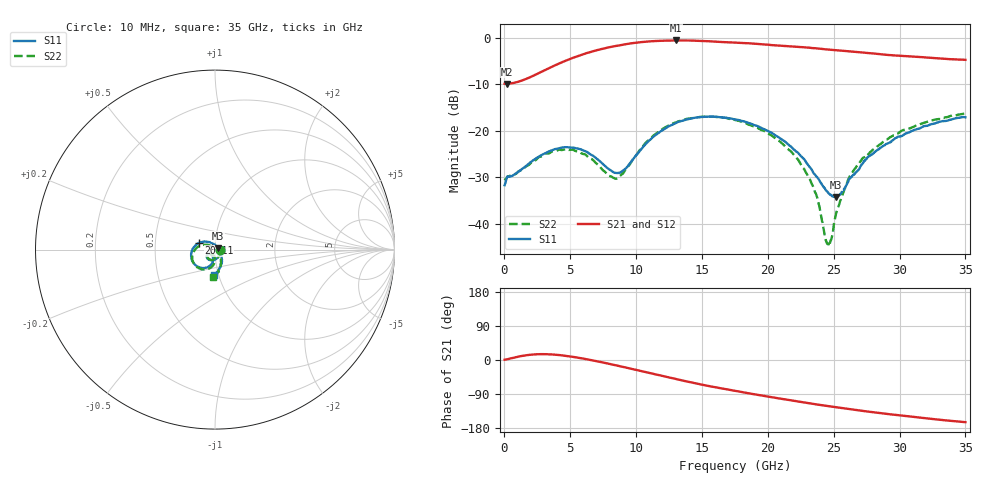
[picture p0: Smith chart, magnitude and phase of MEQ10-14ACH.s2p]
! MARKI MICROWAVE INC.
! Email:  support@markimicrowave.com  Phone:  408-778-4200
! Model Number:  MEQ10-14ACH  Date:  6/18
! Filename:		MEQ10-14ACH.S2P  Version: 1.0
! Description:  2-port S-parameter data for chip equalizer
! Features:		Low Insertion Loss, Excellent Return Loss
! Frequency Measured: 	10 MHz to 35 GHz
!S2P File: Measurements: S11, S21, S12, S22:
# Hz S  dB  R 50
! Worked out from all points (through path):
!   1601 points, 10 MHz to 35 GHz, reference 50 ohm
!   highest |S21| = -0.61 dB at 13 GHz (marker M1); lowest = -9.9 dB at 206.8 MHz (marker M2)
!   group delay of S21, straight-line fit = 16.2 ps
!   lowest |S11| = -34.3 dB at 25.16 GHz (marker M3), VSWR 1.04, Z = 51.7 + j0.915 ohm
!   |S11| at or under -10 dB: start of sweep to end of sweep
!   |S22| runs from -44.9 to -16.3 dB; largest |S21 - S12| = 0.0061
!   S11 on the Smith chart (normalised r, x): 10 MHz: 1.05, -0.00; 20.11 GHz: 0.83, +0.06; 35 GHz: 0.96, -0.27
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1e7  -31.76 -2.9  -9.92 0.7  -9.96 0.0  -30.69 -5.9
2.068188e8  -29.87 -8.5  -9.94 1.9  -9.93 1.8  -29.97 -8.7
3.640212e9  -24.20 -103.7  -6.22 14.6  -6.22 14.6  -24.45 -102.5
5.848956e9  -24.10 -138.2  -3.69 4.5  -3.68 4.5  -24.87 -136.1
8.495075e9  -29.12 -128.2  -1.76 -14.3  -1.75 -14.3  -30.34 -117.5
9.194875e9  -28.18 -110.1  -1.41 -19.8  -1.41 -19.8  -28.34 -97.9
1.168791e10  -20.53 -107.2  -0.70 -40.0  -0.69 -40.0  -20.27 -100.6
1.300004e10  -18.38 -121.6  -0.61 -50.2  -0.60 -50.3  -18.26 -115.1
1.529626e10  -17.03 -148.2  -0.75 -67.1  -0.74 -67.0  -16.98 -141.9
1.7505e10  -17.59 -173.2  -1.06 -81.3  -1.07 -81.5  -17.72 -166.0
2.010738e10  -20.22 157.6  -1.55 -97.4  -1.50 -97.4  -20.80 168.1
2.211931e10  -24.45 133.8  -1.94 -108.5  -1.98 -108.7  -25.69 148.9
2.334396e10  -28.49 113.5  -2.23 -115.3  -2.22 -115.1  -31.50 134.3
2.38032e10  -30.25 100.4  -2.36 -117.8  -2.32 -117.6  -35.04 125.5
2.452487e10  -33.13 69.6  -2.54 -121.4  -2.49 -121.5  -44.41 63.5
2.478729e10  -33.84 53.8  -2.61 -122.8  -2.57 -122.9  -43.62 8.9
2.515906e10  -34.29 27.3  -2.71 -124.6  -2.68 -124.8  -38.15 -24.0
2.642745e10  -29.69 -23.8  -3.01 -130.6  -3.03 -130.7  -28.94 -47.2
2.763023e10  -25.60 -44.1  -3.32 -136.3  -3.31 -136.1  -25.07 -57.0
2.918291e10  -22.66 -58.9  -3.73 -142.8  -3.68 -142.9  -21.67 -66.1
3.18509e10  -19.04 -77.8  -4.23 -153.2  -4.26 -152.9  -18.33 -80.1
3.5e10  -17.15 -91.2  -4.77 -163.9  -4.76 -164.3  -16.31 -93.4
